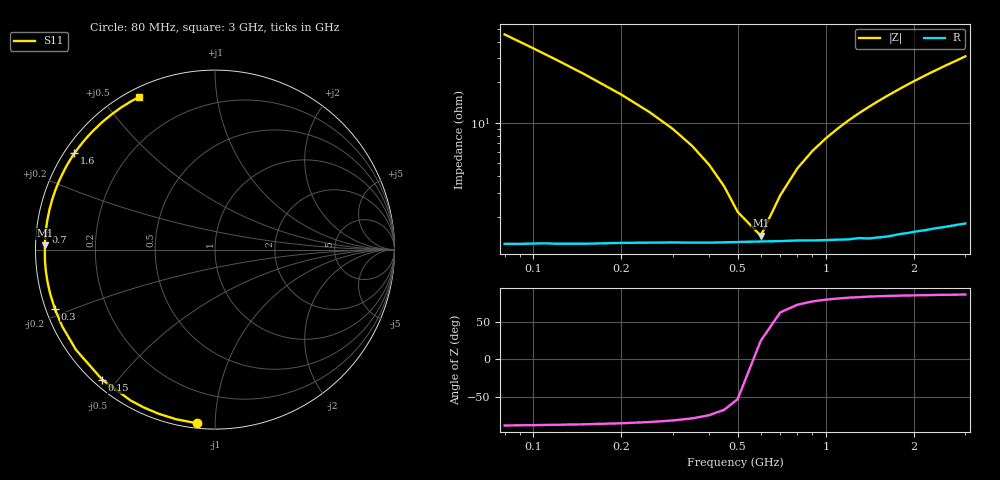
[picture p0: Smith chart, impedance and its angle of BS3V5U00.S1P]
! SIEMENS Small Signal Semiconductors
! BB640
! Si Tuning Diode in SOD323
! VR = 3.5 V
! S-Parameters:  July  1993
# GHz  S  MA  R  50
!  f  S11
! GHz  MAG  ANG
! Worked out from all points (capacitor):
!   33 points, 80 MHz to 3 GHz, reference 50 ohm
!   read as one part to ground: C = 43.2 pF near 80 MHz
!   lowest |Z| = 1.44 ohm at 600 MHz (marker M1)
!   series resonance near 574.1 MHz, so ESL is about 1.8 nH
!   S11 on the Smith chart (normalised r, x): 80 MHz: 0.03, -0.90; 150 MHz: 0.03, -0.46; 300 MHz: 0.03, -0.18; 700 MHz: 0.03, +0.05; 1.6 GHz: 0.03, +0.31; 3 GHz: 0.04, +0.62
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0.08  0.9727 -95.8
0.09  0.9698 -102.8
0.1  0.9671 -108.9
0.11  0.9648 -114.4
0.12  0.9632 -119.2
0.15  0.9592 -130.9
0.2  0.9548 -144.2
0.25  0.9526 -153.2
0.3  0.9513 -159.8
0.35  0.9508 -165.0
0.4  0.9504 -169.3
0.45  0.9499 -172.9
0.5  0.9495 -176.0
0.6  0.949 178.6
0.7  0.9488 174.1
0.8  0.9485 170.0
0.9  0.9488 166.3
1  0.9489 162.9
1.2  0.9493 156.6
1.4  0.9497 150.9
1.6  0.9495 145.6
1.8  0.9486 140.6
2  0.9483 135.9
2.2  0.9484 131.5
2.4  0.9484 127.4
2.6  0.9489 123.5
2.8  0.9492 119.9
3  0.9499 116.3
